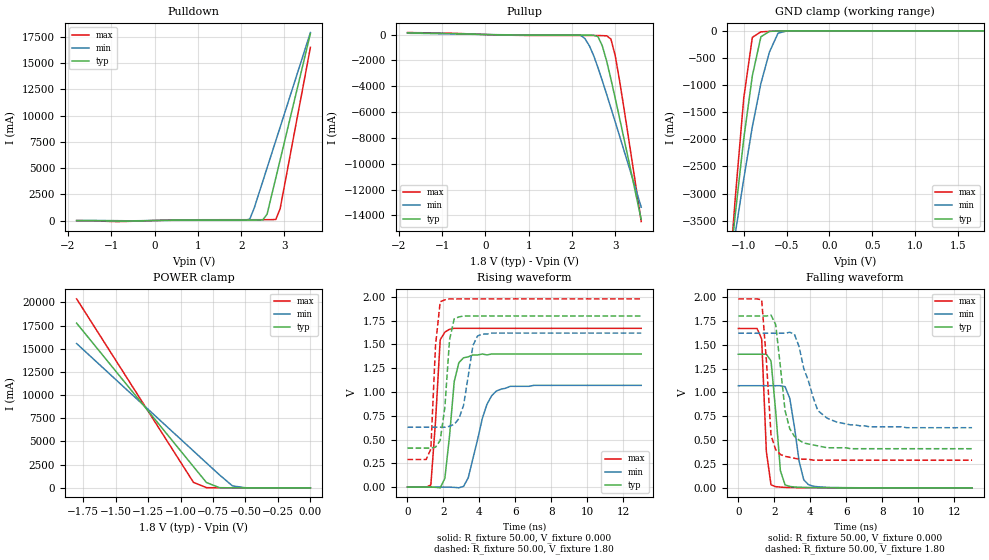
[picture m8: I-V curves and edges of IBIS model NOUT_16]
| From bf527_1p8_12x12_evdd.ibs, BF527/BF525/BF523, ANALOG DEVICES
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|   Model prw1216hcdg_25
[Model]   NOUT_16
Model_type   I/O
Polarity   Non-Inverting
Enable   Active-Low
Vinl =   0.70V
Vinh =   1.00V
Vmeas =   1.20V
Cref =  50.00pF
Rref =   1.00M
Vref =  0.000V
C_comp   4.56pF   4.11pF   5.02pF
[Temperature Range]   25.00   0.12k   -40.00
[Voltage Range]   1.80V   1.62V   1.98V
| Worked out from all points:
|   slope of the pulldown table from 0 to 0.27 V, typ, clamps not added: 13.6 ohm
|   slope of the pullup table from 0 to 0.27 V, typ, clamps not added: 13.3 ohm
|   GND clamp passes 1 mA (typ) near -0.53 V on its own axis
|   POWER clamp passes 1 mA (typ) near -0.53 V on its own axis
|   rising waveform, R_fixture 50.00, V_fixture 0.000: 20-80 % time 424ps typ, 866ps min, 334ps max; typ from 0 V to 1.4 V
|   rising waveform, R_fixture 50.00, V_fixture 1.80: 20-80 % time 363ps typ, 524ps min, 292ps max; typ from 0.41 V to 1.8 V
|   falling waveform, R_fixture 50.00, V_fixture 0.000: 20-80 % time 375ps typ, 535ps min, 245ps max; typ from 1.4 V to 0 V
|   falling waveform, R_fixture 50.00, V_fixture 1.80: 20-80 % time 576ps typ, 941ps min, 359ps max; typ from 1.8 V to 0.41 V
[Pulldown]
| voltage   I(typ)   I(min)   I(max)
-1.8V     -10mA      0A         -10mA
-900mV    -54mA      -13mA      -100mA
600mV     35.42mA    19.28mA    58.01mA
2.1V      42.7mA     29.01mA    73.65mA
2.2V      42.78mA    140mA      73.7mA
2.3V      43.23mA    1.16A      73.76mA
2.5V      59.88mA    3.73A      74.67mA
2.6V      610mA      5.02A      77.38mA
2.8V      4.04A      7.6A       99.24mA
2.9V      5.76A      8.88A      1.1A
3.6V      17.81A     17.91A     16.5A
[Pullup]
| voltage   I(typ)   I(min)   I(max)
-1.8V     130mA      100mA      150mA
2.2V      -46.27mA   -53.72mA   -75.17mA
2.3V      -46.8mA    -320mA     -75.37mA
2.4V      -49mA      -860mA     -75.61mA
2.5V      -56.4mA    -1.62A     -76.58mA
2.6V      -160mA     -2.56A     -80.36mA
2.7V      -870mA     -3.57A     -87.34mA
2.8V      -2.04A     -4.62A     -98.54mA
2.9V      -3.45A     -5.69A     -350mA
3V        -4.95A     -6.77A     -1.65A
3.1V      -6.48A     -7.86A     -3.58A
3.6V      -14.33A    -13.37A    -14.48A
[GND_clamp]
| voltage   I(typ)   I(min)   I(max)
-1.8V     -14.28A    -11.35A    -18.41A
-1.2V     -4.9A      -4.81A     -5.19A
-1.1V     -3.4A      -3.75A     -3.1A
-1V       -1.99A     -2.73A     -1.24A
-900mV    -830mA     -1.77A     -120mA
-800mV    -110mA     -970mA     -19.16mA
-700mV    -9.86mA    -390mA     -9.75mA
-600mV    -2.56mA    -42.82mA   -3.49mA
-500mV    -460uA     -4.35mA    -560uA
1.8V      160pA      3.22uA     -3.16uA
[POWER_clamp]
| voltage   I(typ)   I(min)   I(max)
-1.8V     17.76A     15.56A     20.38A
-900mV    2.28A      3.97A      590mA
-800mV    570mA      2.68A      17mA
-700mV    17.04mA    1.4A       7.09mA
-600mV    2.37mA     210mA      2.78mA
-500mV    460uA      11.86mA    540uA
0V        160pA      7.79nA     87.38pA
[Ramp]
| variable   typ   min   max
dV/dt_r   0.84/0.39n   0.64/0.75n   1.00/0.22n
dV/dt_f   0.83/0.51n   0.59/0.86n   1.01/0.27n
R_load = 50.00
[Rising Waveform]
R_fixture = 50.00
V_fixture = 0.000
V_fixture_min = 0.000
V_fixture_max = 0.000
L_fixture = 0.000H
C_fixture = 0.000F
| time   V(typ)   V(min)   V(max)
0s        0V         0V         0V
1.3ns     -330uV     53.95uV    22.19mV
1.56ns    -2.52mV    42.25uV    690mV
1.82ns    -8.12mV    -26.88uV   1.55V
2.08ns    91.72mV    -360uV     1.63V
2.6ns     1.11V      -3.17mV    1.67V
3.12ns    1.36V      7.73mV     1.67V
4.42ns    1.39V      870mV      1.67V
4.94ns    1.4V       1.01V      1.67V
13ns      1.4V       1.07V      1.67V
[Rising Waveform]
R_fixture = 50.00
V_fixture = 1.80
V_fixture_min = 1.62
V_fixture_max = 1.98
L_fixture = 0.000H
C_fixture = 0.000F
| time   V(typ)   V(min)   V(max)
0s        410mV      630mV      290mV
1.3ns     410mV      630mV      400mV
1.56ns    420mV      630mV      1.49V
1.82ns    490mV      630mV      1.95V
2.08ns    840mV      630mV      1.97V
2.34ns    1.55V      640mV      1.98V
2.6ns     1.77V      660mV      1.98V
3.12ns    1.8V       860mV      1.98V
3.9ns     1.8V       1.59V      1.98V
13ns      1.8V       1.62V      1.98V
[Falling Waveform]
R_fixture = 50.00
V_fixture = 0.000
V_fixture_min = 0.000
V_fixture_max = 0.000
L_fixture = 0.000H
C_fixture = 0.000F
| time   V(typ)   V(min)   V(max)
0s        1.4V       1.07V      1.67V
1.3ns     1.4V       1.07V      1.56V
1.56ns    1.4V       1.07V      380mV
1.82ns    1.33V      1.07V      31.3mV
2.34ns    180mV      1.07V      7.58mV
2.6ns     31.03mV    1.06V      4.94mV
2.86ns    14.76mV    940mV      3.4mV
3.38ns    6.32mV     280mV      1.47mV
3.9ns     3.49mV     34.05mV    830uV
13ns      6.98uV     29.9uV     3.1uV
[Falling Waveform]
R_fixture = 50.00
V_fixture = 1.80
V_fixture_min = 1.62
V_fixture_max = 1.98
L_fixture = 0.000H
C_fixture = 0.000F
| time   V(typ)   V(min)   V(max)
0s        1.8V       1.62V      1.98V
1.3ns     1.8V       1.62V      1.97V
1.82ns    1.81V      1.62V      550mV
2.08ns    1.71V      1.62V      400mV
2.34ns    1.27V      1.62V      350mV
2.86ns    620mV      1.63V      320mV
3.64ns    470mV      1.25V      300mV
4.42ns    440mV      810mV      290mV
5.46ns    420mV      690mV      290mV
13ns      410mV      630mV      290mV
